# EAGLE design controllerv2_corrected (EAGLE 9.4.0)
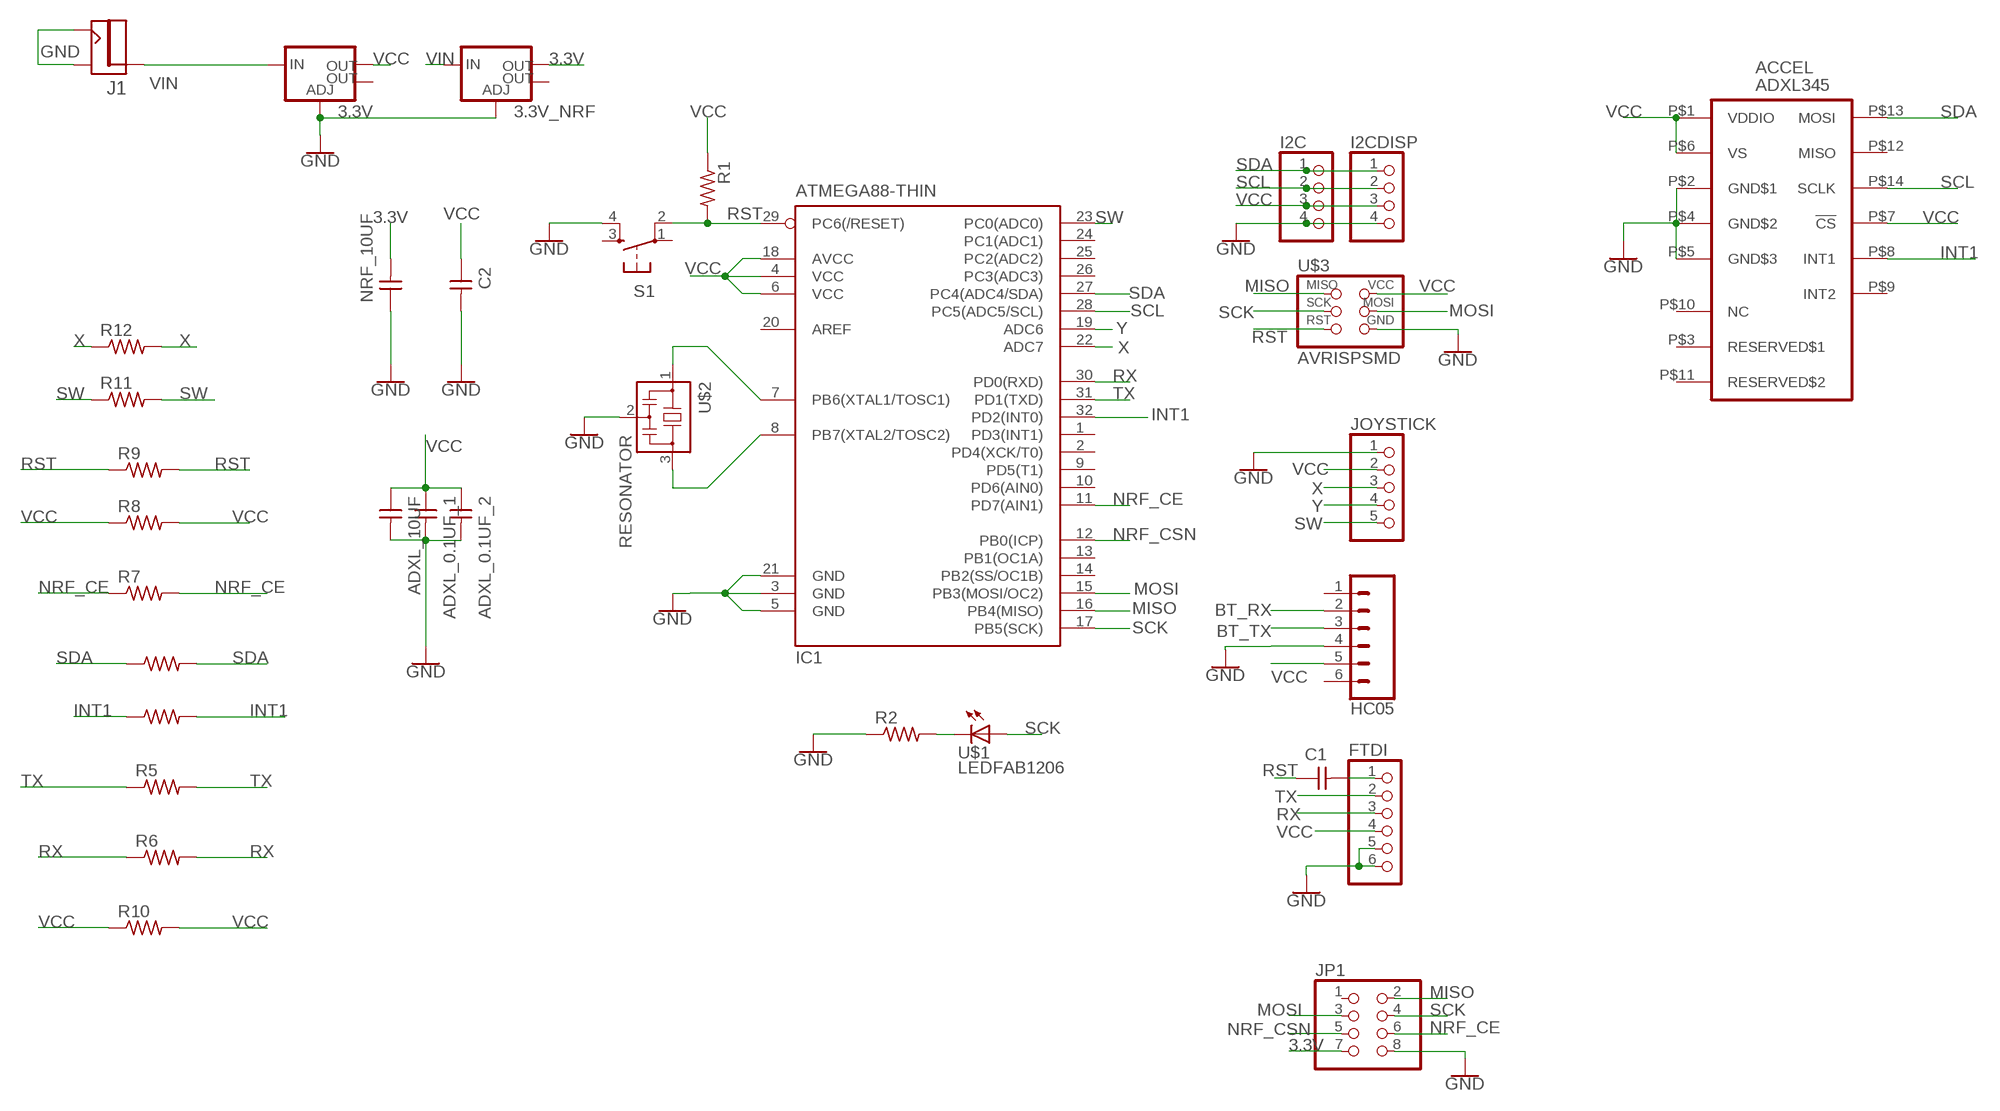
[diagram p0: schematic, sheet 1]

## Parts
3.3V  V_REG_LM1117SOT223  [SOT223]
3.3V_NRF  V_REG_LM1117SOT223  [SOT223]
ACCEL  ADXL345  [LGA14]
ADXL_0.1UF_1  CAP-UNPOLARIZEDFAB  [C1206FAB]
ADXL_0.1UF_2  CAP-UNPOLARIZEDFAB  [C1206FAB]
ADXL_10UF  CAP-UNPOLARIZEDFAB  [C1206FAB]
C1  CAP-UNPOLARIZEDFAB  [C1206FAB]
C2  CAP-UNPOLARIZEDFAB  [C1206FAB]
FTDI  PINHD-1X61X06_SMT  [1X06_SMT]
HC05  CONN_06SMD-FEMALE-V2  [1X06-SMD-FEMALE]
I2C  PINHD-1X41X04_SMT  [1X04_SMT]
I2CDISP  PINHD-1X41X04_SMT  [1X04_SMT]
IC1  ATMEGA88-THIN  [TQFP32-08THIN]
J1  JACK2.1MM  [JACK_2.1MM]
JOYSTICK  PINHD-1X51X05_SMT  [1X05_SMT]
JP1  PINHD-2X4SMT  [2X04_SMT]
NRF_10UF  CAP-UNPOLARIZEDFAB  [C1206FAB]
R1  RES-US1206FAB  [R1206FAB]
R2  RES-US1206FAB  [R1206FAB]
R3  RES-US1206FAB  [R1206FAB]
R4  RES-US1206FAB  [R1206FAB]
R5  RES-US1206FAB  [R1206FAB]
R6  RES-US1206FAB  [R1206FAB]
R7  RES-US1206FAB  [R1206FAB]
R8  RES-US1206FAB  [R1206FAB]
R9  RES-US1206FAB  [R1206FAB]
R10  RES-US1206FAB  [R1206FAB]
R11  RES-US1206FAB  [R1206FAB]
R12  RES-US1206FAB  [R1206FAB]
S1  6MM_SWITCH6MM_SWITCH  [6MM_SWITCH]
U$1  LEDFAB1206  [LED1206FAB]
U$2  RESONATOR  [EFOBM]
U$3  AVRISPSMD  [2X03SMD]

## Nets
3.3V: 3.3V_NRF.2(OUT) JP1.7 NRF_10UF.2
BT_RX: HC05.2
BT_TX: HC05.3
GND: 3.3V.1(ADJ) 3.3V_NRF.1(ADJ) ACCEL.P$2(GND$1) ACCEL.P$4(GND$2) ACCEL.P$5(GND$3) ADXL_0.1UF_1.2 ADXL_0.1UF_2.2 ADXL_10UF.2 C2.2 FTDI.5 FTDI.6 HC05.4 I2C.4 I2CDISP.4 IC1.3(GND) IC1.5(GND) IC1.21(GND) J1.CONTACT J1.SHUNT JOYSTICK.1 JP1.8 NRF_10UF.1 R2.1 S1.4(S1) U$2.2 U$3.6(GND)
INT1: ACCEL.P$8(INT1) IC1.32(PD2(INT0)) R4.1 R4.2
MISO: IC1.16(PB4(MISO)) JP1.2 U$3.1(MISO)
MOSI: IC1.15(PB3(MOSI/OC2)) JP1.3 U$3.4(MOSI)
N$1: IC1.7(PB6(XTAL1/TOSC1)) U$2.1
N$2: IC1.8(PB7(XTAL2/TOSC2)) U$2.3
N$5: C1.2 FTDI.1
N$18: R2.2 U$1.2(C)
NRF_CE: IC1.11(PD7(AIN1)) JP1.6 R7.1 R7.2
NRF_CSN: IC1.12(PB0(ICP)) JP1.5
RST: C1.1 IC1.29(PC6(/RESET)) R1.2 R9.1 R9.2 S1.2(P1) U$3.5(RST)
RX: FTDI.3 IC1.30(PD0(RXD)) R6.1 R6.2
SCK: IC1.17(PB5(SCK)) JP1.4 U$1.1(A) U$3.3(SCK)
SCL: ACCEL.P$14(SCLK) I2C.2 I2CDISP.2 IC1.28(PC5(ADC5/SCL))
SDA: ACCEL.P$13(MOSI) I2C.1 I2CDISP.1 IC1.27(PC4(ADC4/SDA)) R3.1 R3.2
SW: IC1.23(PC0(ADC0)) JOYSTICK.5 R11.1 R11.2
TX: FTDI.2 IC1.31(PD1(TXD)) R5.1 R5.2
VCC: 3.3V.2(OUT) ACCEL.P$1(VDDIO) ACCEL.P$6(VS) ACCEL.P$7(!CS) ADXL_0.1UF_1.1 ADXL_0.1UF_2.1 ADXL_10UF.1 C2.1 FTDI.4 HC05.5 I2C.3 I2CDISP.3 IC1.4(VCC) IC1.6(VCC) IC1.18(AVCC) JOYSTICK.2 R1.1 R8.1 R8.2 R10.1 R10.2 U$3.2(VCC)
VIN: 3.3V.3(IN) 3.3V_NRF.3(IN) J1.PIN
X: IC1.22(ADC7) JOYSTICK.3 R12.1 R12.2
Y: IC1.19(ADC6) JOYSTICK.4
Unconnected: 3.3V.4(OUT) 3.3V_NRF.4(OUT) ACCEL.P$3(RESERVED$1) ACCEL.P$9(INT2) ACCEL.P$10(NC) ACCEL.P$11(RESERVED$2) ACCEL.P$12(MISO) HC05.1 HC05.6 IC1.1(PD3(INT1)) IC1.2(PD4(XCK/T0)) IC1.9(PD5(T1)) IC1.10(PD6(AIN0)) IC1.13(PB1(OC1A)) IC1.14(PB2(SS/OC1B)) IC1.20(AREF) IC1.24(PC1(ADC1)) IC1.25(PC2(ADC2)) IC1.26(PC3(ADC3)) JP1.1 S1.1(P) S1.3(S)

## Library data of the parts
3.3V 3.3V_NRF = fab:V_REG_LM1117: Voltage Regulator LM1117 Standard adjustable voltage regulator but in SMD form. Spark Fun Electronics SKU : COM-00595; PROD_ID: VREG-08170
ACCEL = adxl345:ADXL345: 3-Axis, ±2 g/±4 g/±8 g/±16 g Digital Accelerometer
ADXL_0.1UF_1 ADXL_0.1UF_2 ADXL_10UF C1 C2 NRF_10UF = fab:CAP-UNPOLARIZED
FTDI = smd_con:PINHD-1X6: PIN HEADER
HC05 = SparkFun-Connectors:CONN_06: Multi connection point. Often used as Generic Header-pin footprint for 0.1 inch spaced/style header connections On any of the 0.1 inch spaced packages, you can populate with these: Break Away Headers - Straight (PRT-00116) Break Away Male Headers - Right Angle (PRT-00553) Female Headers (PRT-00115)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; PROD_ID: CONN-09668
I2C I2CDISP = smd_con:PINHD-1X4: PIN HEADER
IC1 = fab:ATMEGA88-THIN
J1 = fab:JACK
JOYSTICK = smd_con:PINHD-1X5: PIN HEADER
JP1 = smd_con:PINHD-2X4: PIN HEADER
R1-R12 = fab:RES-US: Resistor (US Symbol)
S1 = fab:6MM_SWITCH: OMRON SWITCH
U$1 = fab:LED: LED
U$2 = fab:RESONATOR
U$3 = fab:AVRISP

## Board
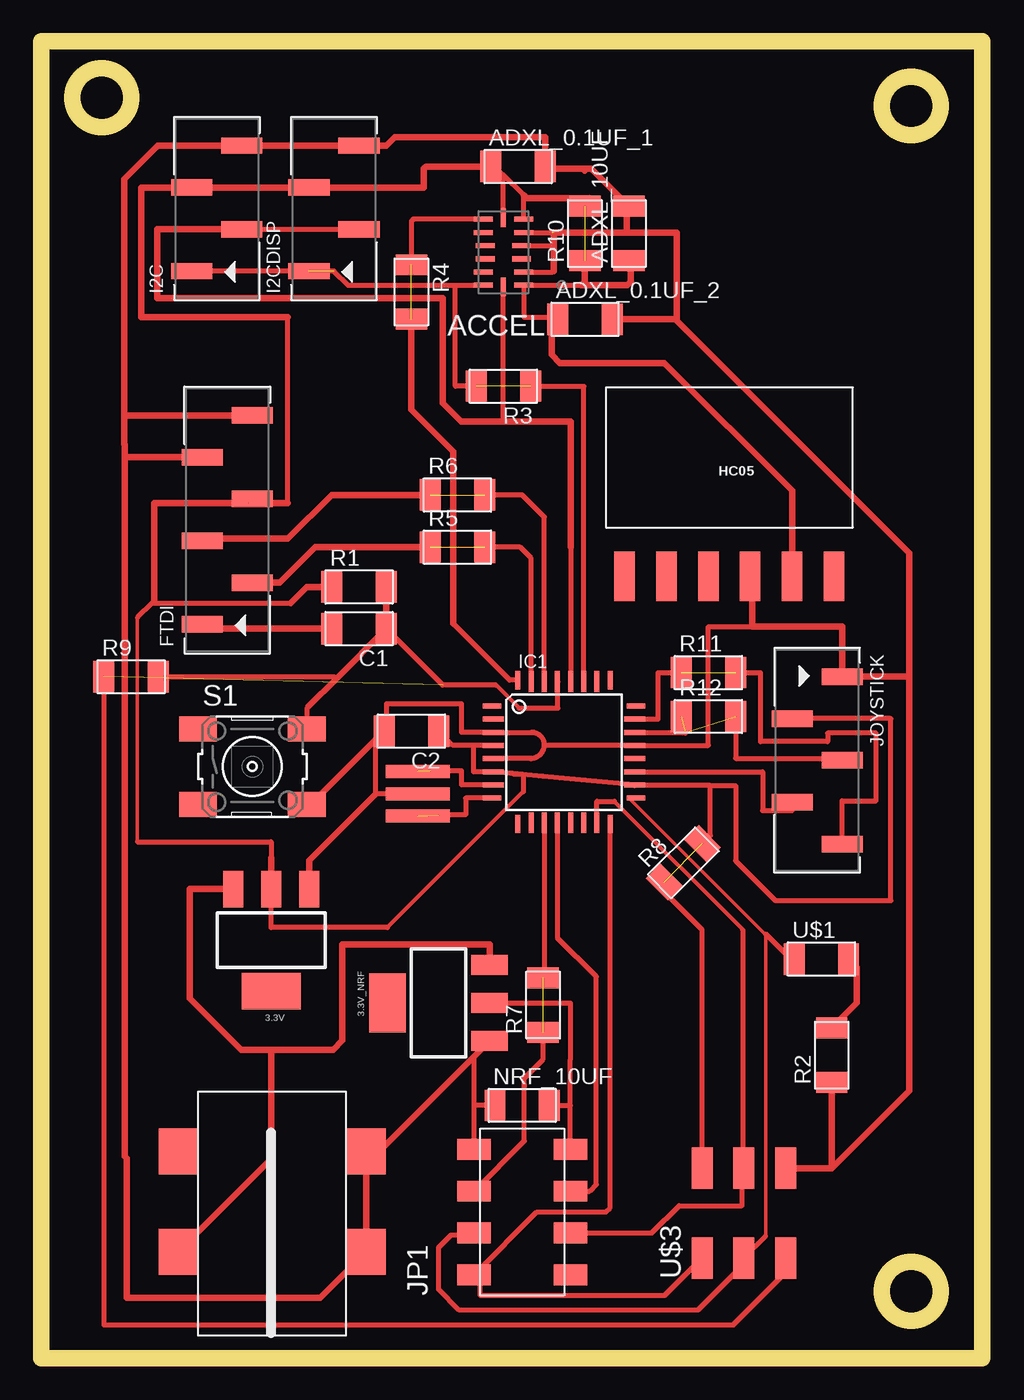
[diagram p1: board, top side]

Size 57.15 x 80.01 mm. Coordinates in mm from the lower left corner, seen from the top.
Outline: 0,80.01 57.15,80.01 57.15,0 0,0 0,80.01
Outline: circle at 52.83,76.07 radius 1.76
Outline: circle at 3.68,76.58 radius 1.76
Outline: circle at 52.83,4.06 radius 1.76
Copper layers (1*16): Top 0.035mm / dielectric 1.5mm / Bottom 0.035mm
Design rules "default *": minimum track width 12mil, minimum drill 0.35mm, track to track 16mil, track to pad 16mil, pad to pad 16mil, via to via 16mil, smd to smd 16mil, copper to edge 40mil, drill to drill 6mil, minimum pad ring 10mil, minimum via ring 8mil, stop-mask expansion 4mil, vias tented up to drill 0mil, thermal gap 10mil

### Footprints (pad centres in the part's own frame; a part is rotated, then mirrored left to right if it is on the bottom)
SOT223 = smd 1.219 x 2.235: 1 -2.311,-3.099; 2 0,-3.099; 3 2.311,-3.099 | smd 3.6 x 2.2: 4 0,3.099
LGA14 = smd 1.15 x 0.305: P$1 -1.227,2; P$2 -1.227,1.2; P$3 -1.1,0.4; P$4 -1.1,-0.4; P$5 -1.227,-1.2; P$6 -1.227,-2; P$8 1.227,-2; P$9 1.227,-1.2; P$10 1.1,-0.4; P$11 1.1,0.4; P$12 1.227,1.2; P$13 1.227,2 | smd 0.305 x 1.15: P$7 0,-2.1; P$14 0,2.1
C1206FAB = smd 1.27 x 1.905: 1 -1.651,0; 2 1.651,0
1X06_SMT = smd 1 x 2.5: 1 -6.35,1.52; 2 -3.81,-1.52; 3 -1.27,1.52; 4 1.27,-1.52; 5 3.81,1.52; 6 6.35,-1.52
1X06-SMD-FEMALE = smd 1.25 x 3: 1 6.35,3.425; 2 3.81,3.425; 3 1.27,3.425; 4 -1.27,3.425; 5 -3.81,3.425; 6 -6.35,3.425
1X04_SMT = smd 1 x 2.5: 1 -3.81,1.52; 2 -1.27,-1.52; 3 1.27,1.52; 4 3.81,-1.52
TQFP32-08THIN = smd 1.118 x 0.305: 1 -4.369,2.8; 8 -4.369,-2.8; 17 4.369,-2.8; 24 4.369,2.8 | smd 1.27 x 0.305: 2 -4.293,2; 3 -4.293,1.2; 4 -4.293,0.4; 5 -4.293,-0.4; 6 -4.293,-1.2; 7 -4.293,-2; 18 4.293,-2; 19 4.293,-1.2; 20 4.293,-0.4; 21 4.293,0.4; 22 4.293,1.2; 23 4.293,2 | smd 0.305 x 1.118: 9 -2.8,-4.369; 16 2.8,-4.369; 25 2.8,4.369; 32 -2.8,4.369 | smd 0.305 x 1.27: 10 -2,-4.293; 11 -1.2,-4.293; 12 -0.4,-4.293; 13 0.4,-4.293; 14 1.2,-4.293; 15 2,-4.293; 26 2,4.293; 27 1.2,4.293; 28 0.4,4.293; 29 -0.4,4.293; 30 -1.2,4.293; 31 -2,4.293
JACK_2.1MM = smd 2.388 x 2.794: CONTACT 5.766,-2.413; PIN -5.639,-2.413; PIN1 -5.639,3.683; SHUNT 5.766,3.683
1X05_SMT = smd 1 x 2.5: 1 -5.08,1.52; 2 -2.54,-1.52; 3 0,1.52; 4 2.54,-1.52; 5 5.08,1.52
2X04_SMT = smd 1.27 x 2.032: 1 -3.81,-2.921; 2 -3.81,2.921; 3 -1.27,-2.921; 4 -1.27,2.921; 5 1.27,-2.921; 6 1.27,2.921; 7 3.81,-2.921; 8 3.81,2.921
R1206FAB = smd 1.27 x 1.905: 1 -1.651,0; 2 1.651,0
6MM_SWITCH = smd 2.286 x 1.524: 1 -3.302,2.286; 2 3.302,2.286; 3 -3.302,-2.286; 4 3.302,-2.286
LED1206FAB = smd 1.27 x 1.905: 1 -1.651,0; 2 1.651,0
EFOBM = smd 0.8 x 3.9: 1 -1.35,0; 2 0,0; 3 1.35,0
2X03SMD = smd 2.54 x 1.27: 1 -2.54,2.54; 2 2.92,2.54; 3 -2.54,0; 4 2.92,0; 5 -2.54,-2.54; 6 2.92,-2.54

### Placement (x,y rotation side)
3.3V  13.97,25.4 180 top
3.3V_NRF  24.13,21.59 90 top
ACCEL  28.07,67.18 180 top
ADXL_0.1UF_1  28.96,72.39 0 top
ADXL_0.1UF_2  33.02,63.12 0 top
ADXL_10UF  35.69,68.33 90 top
C1  19.3,44.32 180 top
C2  22.48,38.1 180 top
FTDI  11.3,50.93 90 top
HC05  41.78,50.93 180 top
I2C  10.67,69.85 90 top
I2CDISP  17.78,69.85 90 top
IC1  31.75,36.83 0 top
J1  13.97,8.89 0 top
JOYSTICK  47.12,36.32 270 top
JP1  29.21,8.89 90 top
NRF_10UF  29.21,15.37 0 top
R1  19.3,46.86 0 top
R2  48.01,18.41 90 top
R3  28.07,59.05 180 top
R4  22.48,64.77 270 top
R5  25.27,49.28 0 top
R6  25.27,52.45 0 top
R7  30.48,21.46 90 top
R8  38.99,30.1 45 top
R9  5.46,41.4 0 top
R10  33.02,68.33 90 top
R11  40.51,41.66 0 top
R12  40.51,38.99 0 top
S1  12.83,35.94 0 top
U$1  47.37,24.26 0 top
U$2  22.86,34.29 270 top
U$3  42.67,8.64 90 top

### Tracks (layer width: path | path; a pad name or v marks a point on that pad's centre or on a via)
3.3V
  Top 0.305: JP1.7 32.13,15.37 | 32.13,15.37 32.13,17.53 32.13,18.16 32.13,21.59 3.3V_NRF.2 26.54,21.59 | NRF_10UF.2 32.13,15.37
GND  (1 unrouted)
  Top 0.305: 19.05,73.66 I2CDISP.4 | ACCEL.P$2 31.06,65.98 31.11,66.04 31.11,67.69 | 31.11,67.69 31.11,68.38 | ACCEL.P$4 31.01,67.58 31.11,67.69 | ACCEL.P$5 30.99,68.38 | 33.02,68.38 33.02,68.43 | 38.61,63.12 ADXL_0.1UF_2.2 | 43.37,47.18 HC05.4 | 30.61,73.28 30.61,73.03 ADXL_0.1UF_1.2 | 12.32,73.66 I2C.4 | 5.08,55.5 5.08,57.28 | 30.54,37.27 arc90 29.79,38.03 IC1.3 25.53,38.03 25.53,39.75 20.96,39.75 20.96,38.1 C2.2 | 30.54,37.27 arc-90 29.7,36.43 IC1.5 | U$2.2 20.32,34.29 20.32,37.59 | 30.54,37.27 30.54,37.23 IC1.21 40.51,37.23 40.51,44.45 43.18,44.45 | JP1.8 26.29,15.37 | 26.29,15.37 26.29,18.34 26.77,18.82 | NRF_10UF.1 26.29,15.37 | 3.3V.1 16.28,27.94 16.51,27.94
  Top 0.406: C2.2 20.32,37.59 16.38,33.66 S1.4 | 19.05,73.66 I2C.4 7.08,73.66 5.05,71.63 5.05,55.53 5.08,55.5 5.08,54.74 | ADXL_0.1UF_1.2 30.73,72.26 32.89,72.26 | 32.89,72.26 33.02,72.14 | 35.56,68.38 33.02,68.38 31.11,68.38 31.11,66.04 | 35.56,68.38 38.61,68.38 38.61,63.12 | FTDI.6 5.08,57.28 | FTDI.5 5.08,54.74 | ADXL_0.1UF_2.2 38.49,63.12 52.7,48.9 52.7,41.4 | 3.3V.1 16.28,30.25 20.32,34.29 | 5.08,54.74 5.08,12.27 5.21,12.14 5.21,3.68 16.94,3.68 J1.CONTACT | 3.3V_NRF.1 26.77,18.82 20.52,12.57 J1.SHUNT J1.CONTACT | U$3.6 48.01,11.56 | 48.01,11.56 52.7,16.25 52.7,41.4 | R2.1 48.01,11.56 | 52.7,41.4 JOYSTICK.1 48.64,44.45 43.18,44.45 43.18,47.5 HC05.4 | I2CDISP.4 20.96,73.66 21.46,74.17 30.61,74.17 30.61,73.03 | 32.89,72.26 33.4,72.26 ADXL_10UF.2 35.56,69.85 35.56,68.38 | 19.74,6.35 J1.CONTACT
INT1  (1 unrouted)
  Top 0.305: ACCEL.P$8 22.64,69.18 22.61,69.22 22.48,69.09 R4.1 | IC1.32 28.44,41.2 25.02,44.62
  Top 0.406: R4.2 22.48,57.63 25.02,55.09 25.02,44.62
MISO
  Top 0.305: U$3.1 37.85,3.81 26.67,3.81 26.67,4.7 JP1.2 30.1,8.89 34.29,8.89 34.55,9.15 IC1.16
MOSI
  Top 0.229: 34.81,33.83 42.6,26.04
  Top 0.305: JP1.3 37.08,7.62 38.73,9.27 42.55,9.27 42.55,11.68 | 34.81,33.83 33.75,33.83 IC1.15 | 42.6,26.04 42.6,11.63 U$3.4 42.55,11.68 | 42.55,11.68 42.55,11.81
N$1  (1 unrouted)
  Top 0.305: IC1.7 25.53,34.83 25.53,35.69 23.62,35.69
N$2  (1 unrouted)
  Top 0.305: IC1.8 25.78,34.03 25.78,33.02 24.13,33.02
N$5
  Top 0.305: 10.16,44.32 10.04,44.32 FTDI.1
  Top 0.406: C1.2 10.16,44.32
N$18
  Top 0.305: 49.15,24.13 U$1.2
  Top 0.406: R2.2 49.53,21.59 49.53,23.75 U$1.2
NRF_CE  (1 unrouted)
  Top 0.305: JP1.6 29.34,13.21 29.34,16.51 29.34,16.64 29.34,17.02 30.48,18.16 R7.1 | IC1.11 30.55,23.18 R7.2
NRF_CSN
  Top 0.305: JP1.5 33.3,10.16 33.71,10.56 33.71,23.19 31.35,25.55 IC1.12
RST  (1 unrouted)
  Top 0.229: 27.63,40.89 29.02,39.5
  Top 0.305: C1.1 24.38,40.89 27.63,40.89 | 29.02,39.5 31.37,39.5 31.37,41.1 IC1.29 | 16.26,39.62 16.13,39.5 S1.2 | R9.2 17.78,41.4 17.91,41.27 | U$3.5 45.21,5.71 45.47,5.46 42.04,2.03 3.81,2.03 R9.1
  Top 0.406: R1.2 C1.1 17.91,41.27 16.26,39.62
RX  (1 unrouted)
  Top 0.305: IC1.30 30.55,51.11 29.21,52.45 R6.2
  Top 0.406: FTDI.3 9.91,49.78 14.99,49.78 17.65,52.45 R6.1
SCK
  Top 0.203: 35.69,34.03 43.99,25.73 | 43.99,25.73 43.99,25.65 43.99,7.42 | 43.99,25.78 43.99,25.73
  Top 0.305: IC1.17 35.69,34.03 | 45.59,24.38 U$1.1 | U$1.1 45.72,23.59 | JP1.4 26.16,7.49 24.89,7.49 24.13,6.73 24.13,4.19 25.4,2.92 39.88,2.92 42.67,5.71 U$3.3 43.99,7.42 | U$1.1 45.52,24.26 43.99,25.78
SCL
  Top 0.305: I2C.2 I2CDISP.2 | 32.15,49.28 IC1.28 | ACCEL.P$14 28.07,56.9 25.82,56.9 | 7.09,66.77 7.09,64.39
  Top 0.406: I2C.2 7.04,68.58 7.04,64.39 7.09,64.39 24.38,64.39 24.38,58.02 25.51,56.9 25.82,56.9 32.15,56.9 32.15,49.28
SDA  (2 unrouted)
  Top 0.305: I2C.1 17.78,66.04 18.64,65.18 25.15,65.18 | 25.15,65.18 ACCEL.P$13 | IC1.27 32.95,59.05 R3.1 | R3.2 25.15,59.05 25.15,65.18
SW  (1 unrouted)
  Top 0.305: IC1.23 37.47,38.83 37.47,41.66 R11.1 | R11.2 43.69,41.66 43.69,37.46 47.75,37.46 47.75,37.97 50.7,37.97 50.7,33.87 48.64,33.87 JOYSTICK.5
TX  (1 unrouted)
  Top 0.305: IC1.31 29.75,48.61 29.08,49.28 R5.2
  Top 0.406: R5.1 16.64,49.28 14.48,47.12 FTDI.2
VCC  (5 unrouted)
  Top 0.203: 5.84,44.99 5.84,31.37
  Top 0.229: 29.29,34.43 21.01,26.16
  Top 0.305: 10.03,71.12 I2C.3 | 30.86,63.25 29.34,63.25 29.29,63.29 ACCEL.P$1 32.8,65.18 32.89,65.28 | 30.86,63.25 31.5,63.25 31.75,63.5 | ACCEL.P$6 29.29,70.66 28.07,71.88 | ADXL_0.1UF_1.1 27.56,72.39 28.07,71.88 | 31.5,62.36 31.37,62.48 ADXL_0.1UF_2.1 | 30.99,60.96 30.99,63.12 30.86,63.25 | I2CDISP.3 17.27,71.12 | 14.99,51.94 14.99,63.25 | 12.57,51.94 12.7,52.07 | 6.73,45.88 15.15,45.88 | IC1.4 26.29,37.23 | 26.29,37.23 25,37.23 C2.1 | 26.29,37.23 26.29,37.14 26.26,37.14 26.26,35.63 IC1.6 28.5,35.53 28.65,35.52 | 28.65,35.52 29.29,35.46 29.29,34.43 | 40.64,34.8 36.04,34.8 IC1.18 30.46,35.35 29.2,35.47 28.7,35.47 28.65,35.52 | 21.01,26.16 13.97,26.16 3.3V.2 13.97,29.21 | R8.2 40.64,31.75 40.64,34.8 | U$3.2 40.13,26.03 37.82,28.34 R8.1 | 6.86,46.01 6.73,45.88 | 6.73,45.88 5.84,44.99 | 5.84,31.37 13.97,31.37 13.97,29.84 | 40.64,34.8 42.16,34.8 42.16,30.23 44.58,27.81 51.59,27.81 51.59,38.86 JOYSTICK.2 | ACCEL.P$7 28.07,71.88
  Top 0.406: 14.99,51.94 12.57,51.94 | 14.99,63.25 6.07,63.25 6.07,71.12 I2C.3 | ADXL_0.1UF_1.1 23.37,72.39 23.24,72.26 23.24,71.12 17.27,71.12 | I2CDISP.3 10.03,71.12 | ADXL_0.1UF_2.1 30.99,62.74 30.99,60.96 31.5,60.45 37.85,60.45 45.59,52.7 HC05.5 | FTDI.4 12.57,51.94 6.86,51.94 6.86,46.01 | R1.1 16.13,46.86 15.15,45.88 | 13.97,29.21 13.97,29.84 13.97,30.4 | 32.8,65.18 35.59,65.18 35.81,65.41 35.81,66.55 ADXL_10UF.1 | 29.29,70.66 29.46,70.48 33.27,70.48 33.27,70.23 R10.2 | R10.1 33.02,65.41 32.89,65.28
VIN
  Top 0.406: 3.3V.3 9.02,28.5 9.02,21.86 12.15,18.73 13.97,18.73 | 13.97,18.73 17.72,18.73 18.29,19.3 18.29,25.15 27.23,25.15 3.3V_NRF.3 | J1.PIN 13.97,12.12 13.97,18.73
X  (2 unrouted)
  Top 0.305: IC1.22 39.12,38.03 39.12,37.97 | R12.2 42.16,36.45 48.64,36.45 JOYSTICK.3
Y
  Top 0.305: IC1.19 43.81,35.63 43.81,33.27 45.6,33.27 JOYSTICK.4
